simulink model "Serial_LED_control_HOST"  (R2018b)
settings: Solver=VariableStepAuto  StartTime=0.0  StopTime=inf  RelTol=1e-3
undefined symbols (not defined in the file): COM
libraries: c2000scilib x3

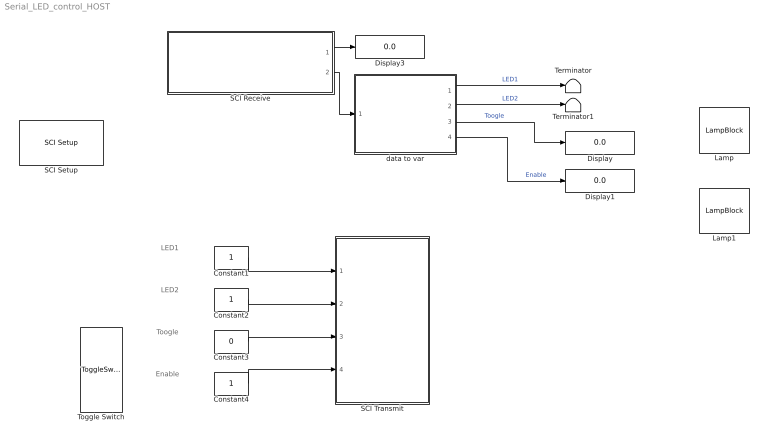
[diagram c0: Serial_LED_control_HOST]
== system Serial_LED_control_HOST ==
  note: LED1
  note: LED2
  note: Toogle
  note: Enable
  Constant1 : Constant  OutMin=[0]  OutMax=[1]  OutDataTypeStr=boolean
  Constant2 : Constant  OutMin=[0]  OutMax=[1]  OutDataTypeStr=boolean
  Constant3 : Constant  Value=0  OutDataTypeStr=boolean
  Constant4 : Constant  OutDataTypeStr=boolean
  Display : Display
  Display1 : Display
  Display3 : Display
  Lamp : LampBlock  WebBlockId=209
  Lamp1 : LampBlock  WebBlockId=211
  SCI Receive : Subsystem
  SCI Setup : c2000scilib/SCI Setup  Priority=-99  commModeA=raw data  baudRateA=115200  charLenA=8  stopBitA=1  parityA=none  timeoutA=1.0  commModeB=raw data  baudRateB=115200  charLenB=8  stopBitB=1  parityB=none  timeoutB=1.0  commModeC=raw data  baudRateC=115200  charLenC=8  stopBitC=1  parityC=none  timeoutC=1.0  commModeD=raw data  baudRateD=115200  charLenD=8  stopBitD=1  parityD=none  timeoutD=1.0
  SCI Transmit : Subsystem
  Terminator : Terminator
  Terminator1 : Terminator
  Toggle Switch : ToggleSwitchBlock  WebBlockId=195  LabelPosition=Hide
  data to var : Subsystem
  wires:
  SCI Receive/1(SCI Status) -> Display3/1
  Constant1/1 -> SCI Transmit/1(LED1)
  Constant2/1 -> SCI Transmit/2(LED2)
  Constant3/1 -> SCI Transmit/3(ToogleLED)
  SCI Receive/2(data) -> data to var/1(data in)
  Constant4/1 -> SCI Transmit/4(Enable)
  data to var/1(LED1) -> Terminator/1  "LED1"
  data to var/2(LED2) -> Terminator1/1  "LED2"
  data to var/3(Toogle) -> Display/1  "Toogle"
  data to var/4(Enable) -> Display1/1  "Enable"

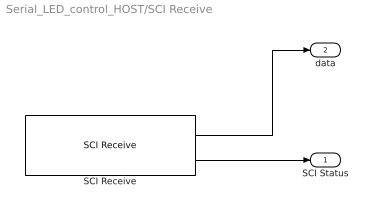
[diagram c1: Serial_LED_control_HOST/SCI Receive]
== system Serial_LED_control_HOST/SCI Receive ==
  SCI Receive : c2000scilib/SCI Receive  module=COM 4  dataHead='S'  dataTail='E'  dataType=uint8  dataDim=4  initValue=0  errOption=Output the last received value  errValue=0  sampleTime=0.1  outputStatus=on
  SCI Status : Outport
  data : Outport  Port=2
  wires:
  SCI Receive/2 -> SCI Status/1
  SCI Receive/1 -> data/1

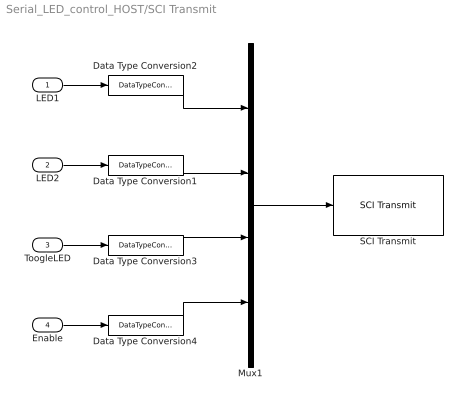
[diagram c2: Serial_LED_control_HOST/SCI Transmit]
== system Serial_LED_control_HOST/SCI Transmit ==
  LED1 : Inport
  LED2 : Inport  Port=2
  ToogleLED : Inport  Port=3
  Enable : Inport  Port=4
  Data Type Conversion{1..4} (4 alike) : DataTypeConversion  OutDataTypeStr=uint8
  Mux1 : Mux
  SCI Transmit : c2000scilib/SCI Transmit  module=COM 4  header='S'  tail='E'
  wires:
  Mux1/1 -> SCI Transmit/1
  LED1/1 -> Data Type Conversion2/1
  LED2/1 -> Data Type Conversion1/1
  Enable/1 -> Data Type Conversion4/1
  ToogleLED/1 -> Data Type Conversion3/1
  Data Type Conversion2/1 -> Mux1/1
  Data Type Conversion1/1 -> Mux1/2
  Data Type Conversion3/1 -> Mux1/3
  Data Type Conversion4/1 -> Mux1/4

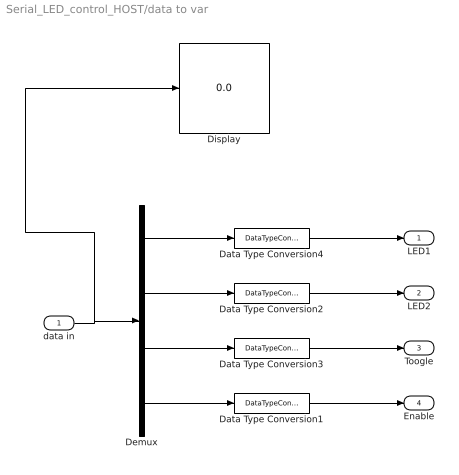
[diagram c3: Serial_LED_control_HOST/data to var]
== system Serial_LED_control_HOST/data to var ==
  data in : Inport
  Data Type Conversion{1..4} (4 alike) : DataTypeConversion  OutDataTypeStr=boolean
  Demux : Demux
  Display : Display
  LED1 : Outport
  LED2 : Outport  Port=2
  Toogle : Outport  Port=3
  Enable : Outport  Port=4
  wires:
  data in/1 -> Display/1, Demux/1
  Data Type Conversion3/1 -> Toogle/1
  Demux/3 -> Data Type Conversion3/1
  Demux/1 -> Data Type Conversion4/1
  Demux/2 -> Data Type Conversion2/1
  Demux/4 -> Data Type Conversion1/1
  Data Type Conversion1/1 -> Enable/1
  Data Type Conversion2/1 -> LED2/1
  Data Type Conversion4/1 -> LED1/1
